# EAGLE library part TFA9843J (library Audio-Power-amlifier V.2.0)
The TFA9843J contains two identical audio power amplifiers. The TFA9843J can be used as two Single-Ended (SE) channels with a fixed gain of 26 dB or one Bridge-Tied Load (BTL) channel with a fixed gain of 32 dB. The TFA9843J comes in a 9-pin DIL-bent-SIL (DBS7P) power package. The TFA9843J is pin compatible with the TFA9842J and TFA9841J. The TFA9843J contains a unique protection circuit that is solely based on multiple temperature measurements inside the chip. This gives maximum output power for all supply voltages and load conditions with no unnecessary audio holes. Almost any supply voltage and load impedance combination can be made as long as thermal boundary conditions (number of channels used, external heatsink and ambient temperature) allow it.
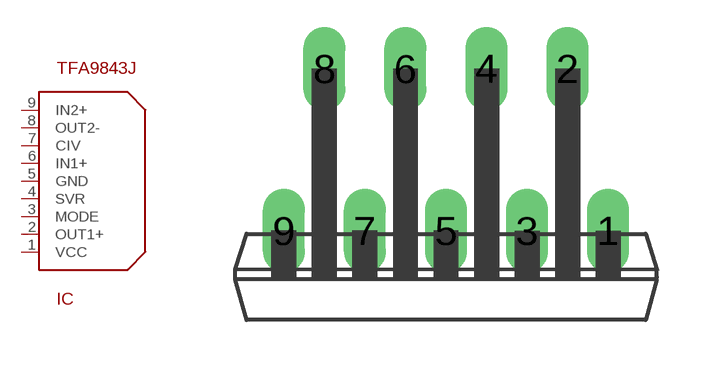
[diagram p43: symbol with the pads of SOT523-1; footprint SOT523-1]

Designator prefix IC

## TFA9843J  [SOT523-1]
1  VCC  pwr
2  OUT1+  out
3  MODE
4  SVR
5  GND  pwr
6  IN1+  in
7  CIV
8  OUT2-  out
9  IN2+  in

## Footprint SOT523-1 (pad centres in mm)
drill 0.8 long: 1 5.08,0; 2 3.81,5.08; 3 2.54,0; 4 1.27,5.08; 5 0,0; 6 -1.27,5.08; 7 -2.54,0; 8 -3.81,5.08; 9 -5.08,0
